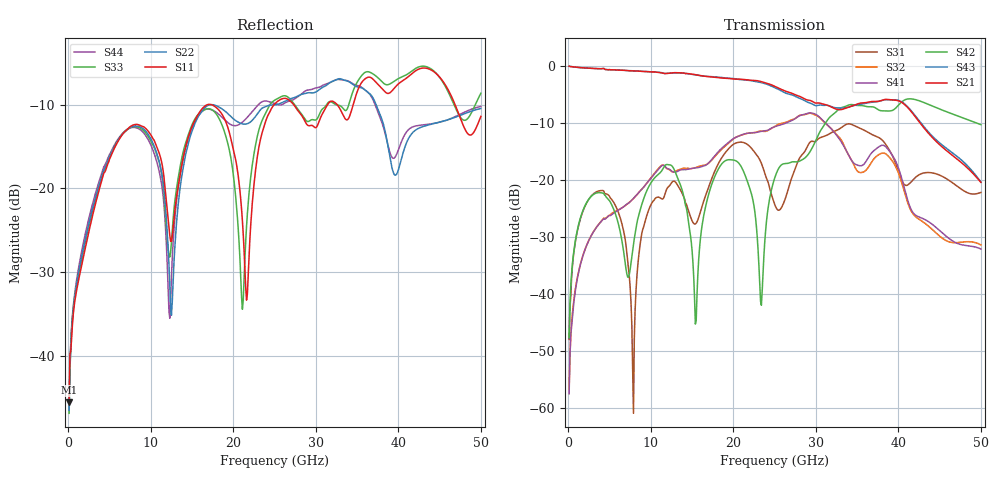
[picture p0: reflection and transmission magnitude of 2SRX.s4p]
! DAC39RF10ACK
! 256-pin FCBGA package
! Texas Instruments 8/20/2022
! Single-ended  S-parameters
! PORT#  PORT_NAME  NET_NAME
! PORT1:  xSRXN.DIEBUMP  xSRXN
! PORT2:  xSRXN.BGA  xSRXN
! PORT3:  xSRXP.DIEBUMP  xSRXP
! PORT4:  xSRXP.BGA  xSRXP
! Touchstone Ver. 1.0
! Number of ports is 4
# Hz	S	MA	R	50.000000
! SCATTERING PARAMETERS  :
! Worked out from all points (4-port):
!   500 points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, 100 MHz to 50 GHz, reference 50 ohm
!   strongest paths, dB at 100 MHz, 12.6 GHz, 25.1 GHz, 37.6 GHz, 50 GHz:
!     S21: 0.0, -1.2, -3.6, -6.2, -20.4
!     S43: 0.0, -1.2, -3.9, -6.2, -20.3
!     S42: -47.7, -17.6, -19.3, -7.7, -10.3
!     S41: -57.5, -18.5, -10.6, -14.2, -32.1
!     S32: -56.7, -18.6, -10.5, -15.6, -31.4
!     S31: -48.0, -20.3, -24.6, -12.5, -22.2
!   lowest |S11| = -45.5 dB at 100 MHz (marker M1), VSWR 1.01, Z = 50.4 + j0.358 ohm
!   |S11| at or under -10 dB: start of sweep to 16.86 GHz; 17.33 GHz to 24.94 GHz (7.613 GHz wide, 36 % of centre); 27.31 GHz to 31.42 GHz (4.109 GHz wide, 14 % of centre)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
1e8  0.005301 42.1  0.9958 -2.5  0.003798 84.3  0.001433 -99.0
     0.9957 -2.6  0.004745 37.1  0.001317 -98.4  0.004107 83.4
     0.004003 81.7  0.00146 -99.2  0.004549 38.3  0.9958 -2.5
     0.001334 -96.2  0.00414 83.4  0.9961 -2.5  0.004894 38.4
4.1e9  0.1136 15.0  0.9468 -92.1  0.08092 -6.8  0.04376 164.5
       0.9467 -92.0  0.1194 -33.8  0.04467 164.3  0.07663 -3.6
       0.08085 -6.9  0.04449 164.4  0.1189 16.0  0.9445 -92.9
       0.04423 164.7  0.07692 -3.5  0.9474 -92.8  0.1253 -35.6
7.9e9  0.2394 -63.4  0.9043 -175.7  0.0008229 115.6  0.06867 92.8
       0.9057 -175.6  0.2349 -109.8  0.0687 91.4  0.02713 139.0
       0.0009 95.5  0.0689 91.6  0.2337 -63.0  0.9036 -177.2
       0.06896 92.6  0.02736 139.6  0.9074 -177.1  0.2314 -112.8
1.57e10  0.2742 -80.2  0.8314 11.0  0.04718 163.3  0.129 -83.7
         0.8299 10.8  0.2657 -81.2  0.13 -86.0  0.01367 90.3
         0.04471 162.5  0.1306 -86.1  0.2751 -80.3  0.8296 8.1
         0.1283 -84.1  0.01486 94.9  0.8311 7.9  0.2683 -86.9
1.99e10  0.1797 -163.9  0.7697 -81.1  0.2023 9.3  0.2273 -171.6
         0.7699 -81.3  0.263 -129.8  0.2259 -173.8  0.1507 22.4
         0.203 9.1  0.2262 -173.6  0.1316 -170.7  0.7763 -86.1
         0.228 -171.6  0.1501 22.2  0.7774 -86.0  0.238 -123.9
2.35e10  0.2157 -42.0  0.7256 -165.0  0.1347 -109.1  0.2677 93.9
         0.7249 -165.0  0.3015 -125.0  0.269 90.9  0.01135 75.1
         0.1341 -110.6  0.2679 89.5  0.2553 -45.1  0.7106 -170.5
         0.2681 94.0  0.01073 64.0  0.7107 -170.4  0.3295 -126.6
5e10  0.2692 -102.4  0.108 7.4  0.06878 -134.8  0.02737 -124.6
      0.09539 13.4  0.3001 -138.0  0.02586 -104.9  0.3097 -28.7
      0.07782 -138.0  0.027 -115.9  0.3704 -104.6  0.108 -4.7
      0.02482 -116.9  0.3059 -29.0  0.09625 -4.6  0.3086 -137.3
